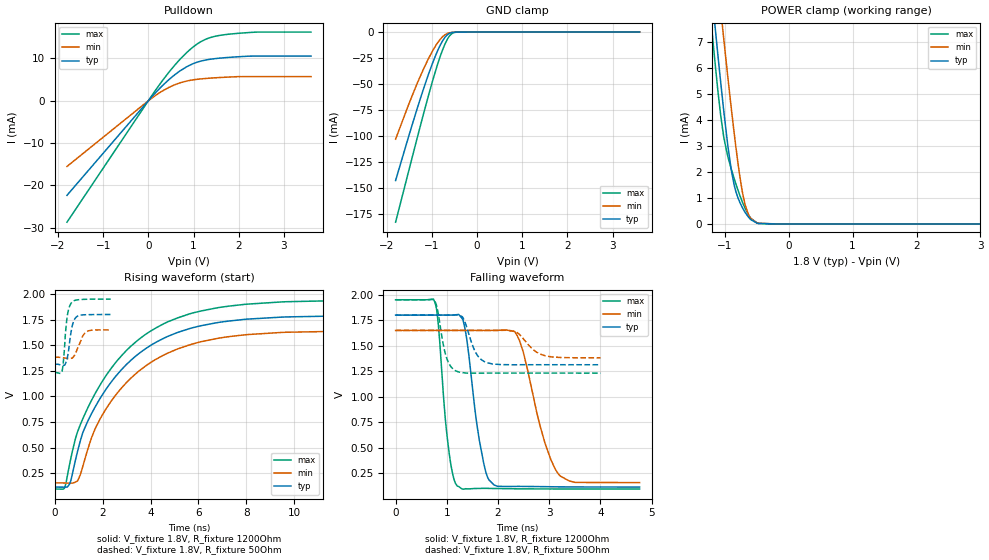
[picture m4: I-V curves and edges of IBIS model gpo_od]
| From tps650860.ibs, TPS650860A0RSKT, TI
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|   gpo_od Model
[Model]   gpo_od
Model_type   Open_drain
Polarity   Non-Inverting
Vmeas = 0.9
Vref = 1.8
Cref = 2pF
Rref = 1200
|   typ   min   max
|   (nom PVT)   (fast PVT)   (slow PVT)
C_comp   1.073e-12   8.143e-13   1.258e-12
| Where nom  PVT is Nominal Process, 1.8V, 27C
|   Fast PVT is Strong Process,  1.95V, -40C
|   Slow PVT is Weak Process,   1.65V, 125C
[Voltage Range]   1.8   1.65   1.95
|Junction Temperature
[Temperature Range]   27   125   -40
[Pullup Reference]   1.8   1.65   1.95
[Pulldown Reference]   0   0   0
[Power Clamp Reference]   1.8   1.65   1.95
[GND Clamp Reference]   0   0   0
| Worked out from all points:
|   slope of the pulldown table from 0 to 0.27 V, typ, clamps not added: 86.2 ohm
|   GND clamp passes 1 mA (typ) near -0.60 V on its own axis
|   POWER clamp passes 1 mA (typ) near -0.79 V on its own axis
|   falling waveform, V_fixture 1.8V, R_fixture 1200Ohm: 20-80 % time 265ps typ, 445ps min, 185ps max; typ from 1.8 V to 0.117 V
|   rising waveform, V_fixture 1.8V, R_fixture 1200Ohm: 20-80 % time 2.84ns typ, 2.81ns min, 2.9ns max; typ from 0.116 V to 1.8 V
|   falling waveform, V_fixture 1.8V, R_fixture 50Ohm: 20-80 % time 216ps typ, 312ps min, 165ps max; typ from 1.8 V to 1.31 V
|   rising waveform, V_fixture 1.8V, R_fixture 50Ohm: 20-80 % time 193ps typ, 291ps min, 165ps max; typ from 1.31 V to 1.8 V
[Pulldown]
|   Voltage   I(typ)   I(min)   I(max)
-1.8V     -22.35mA   -15.52mA   -28.7mA
178.2mV   2.121mA    1.402mA    2.787mA
450.3mV   4.953mA    3.13mA     6.675mA
588.7mV   6.18mA     3.802mA    8.46mA
850mV     8.042mA    4.67mA     11.4mA
1.006V    8.834mA    4.97mA     12.84mA
1.17V     9.399mA    5.178mA    14.01mA
1.33V     9.749mA    5.324mA    14.8mA
1.548V    10.04mA    5.476mA    15.4mA
1.764V    10.24mA    5.599mA    15.72mA
2.418V    10.56mA    5.709mA    16.24mA
3.6V      10.56mA    5.709mA    16.24mA
[GND Clamp]
|   Voltage   I(typ)   I(min)   I(max)
-1.8V     -142.8mA   -103mA     -182.8mA
-1.508V   -99.95mA   -69.36mA   -133.3mA
-1.334V   -75.24mA   -50.66mA   -103.9mA
-1.19V    -55.66mA   -36.29mA   -79.98mA
-984.9mV  -30.23mA   -18.39mA   -47.53mA
-874.8mV  -18.43mA   -10.56mA   -31.57mA
-753.9mV  -7.997mA   -4.213mA   -16.44mA
-648.3mV  -2.341mA   -1.23mA    -6.432mA
-554mV    -416.9uA   -272.7uA   -1.458mA
-458.4mV  -41.96uA   -40.52uA   -138.2uA
-180mV    0A         -40.93nA   0A
3.6V      0A         0A         0A
[POWER Clamp]
|   Voltage   I(typ)   I(min)   I(max)
-1.8V     24.73mA    26.85mA    24.69mA
-1.251V   10.1mA     12.83mA    8.8mA
-1.175V   8.159mA    10.94mA    6.768mA
-1.114V   6.645mA    9.45mA     5.26mA
-1.02V    4.443mA    7.216mA    3.41mA
-950.4mV  2.982mA    5.61mA     2.577mA
-849.6mV  1.463mA    3.426mA    1.719mA
-716.4mV  591.3uA    1.124mA    795.9uA
-592.9mV  165.6uA    205.8uA    217.9uA
-471.8mV  17.65uA    26.36uA    18.44uA
-180mV    0A         39.55nA    0A
3.6V      0A         0A         0A
[Ramp]
R_load = 1200
|   typ   min   max
dV/dt_r   1.01038/2.83708e-09   0.895861/2.80349e-09   1.11161/2.90008e-09
dV/dt_f   1.01039/2.62653e-10   0.895898/4.40994e-10   1.11161/1.84926e-10
[Falling Waveform]
V_fixture = 1.8V
V_fixture_min = 1.65V
V_fixture_max = 1.95V
R_fixture = 1200Ohm
|   Time   V(typ)   V(min)   V(max)
0s        1.8V       1.65V      1.95V
766ps     1.8V       1.65V      1.928V
1.016ns   1.8V       1.65V      569.5mV
1.204ns   1.805V     1.65V      126.6mV
1.366ns   1.637V     1.65V      100.8mV
1.728ns   333.1mV    1.65V      104mV
1.92ns    138.1mV    1.65V      102.7mV
2.374ns   123.4mV    1.6V       99.67mV
3.214ns   118.8mV    225.1mV    98.14mV
4.764ns   116.6mV    160.4mV    98.07mV
[Rising Waveform]
V_fixture = 1.8V
V_fixture_min = 1.65V
V_fixture_max = 1.95V
R_fixture = 1200Ohm
|   Time   V(typ)   V(min)   V(max)
0s        116mV      156.8mV    97.31mV
402ps     114.9mV    155.9mV    103.4mV
658ps     168.9mV    154.4mV    381.9mV
952ps     464.8mV    176.3mV    655.1mV
1.668ns   890.2mV    674.9mV    1.021V
2.252ns   1.107V     918.7mV    1.241V
3.462ns   1.409V     1.237V     1.547V
5.11ns    1.623V     1.462V     1.765V
9.48ns    1.774V     1.624V     1.922V
20ns      1.8V       1.65V      1.95V
[Falling Waveform]
V_fixture = 1.8V
V_fixture_min = 1.65V
V_fixture_max = 1.95V
R_fixture = 50Ohm
|   Time   V(typ)   V(min)   V(max)
0s        1.8V       1.65V      1.95V
744ps     1.8V       1.65V      1.952V
1.004ns   1.8V       1.65V      1.37V
1.218ns   1.803V     1.65V      1.246V
1.34ns    1.749V     1.65V      1.235V
1.566ns   1.432V     1.65V      1.232V
1.778ns   1.335V     1.65V      1.232V
2.35ns    1.314V     1.637V     1.232V
2.918ns   1.314V     1.402V     1.232V
4ns       1.314V     1.382V     1.232V
[Rising Waveform]
V_fixture = 1.8V
V_fixture_min = 1.65V
V_fixture_max = 1.95V
R_fixture = 50Ohm
|   Time   V(typ)   V(min)   V(max)
0s        1.314V     1.382V     1.232V
304ps     1.304V     1.379V     1.245V
372ps     1.303V     1.377V     1.371V
440ps     1.317V     1.374V     1.598V
518ps     1.37V      1.372V     1.777V
586ps     1.464V     1.37V      1.857V
698ps     1.653V     1.373V     1.914V
898ps     1.775V     1.437V     1.941V
1.292ns   1.797V     1.624V     1.948V
2.336ns   1.8V       1.649V     1.95V
